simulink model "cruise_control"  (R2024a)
settings: Solver=VariableStepAuto  StartTime=0.0  StopTime=100  RelTol=1e-3
undefined symbols (not defined in the file): b, m

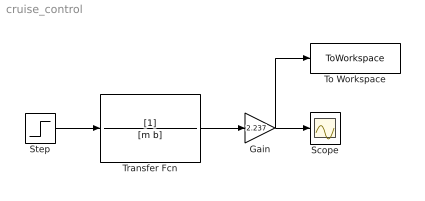
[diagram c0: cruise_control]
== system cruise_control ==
  Gain : Gain  Gain=2.237
  Scope : Scope
  Step : Step  Time=0  After=u  SampleTime=0
  To Workspace : ToWorkspace  VariableName=speed  SaveFormat=Timeseries  SampleTime=-1
  Transfer Fcn : TransferFcn  Denominator=[m b]
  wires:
  Step/1 -> Transfer Fcn/1
  Gain/1 -> To Workspace/1, Scope/1
  Transfer Fcn/1 -> Gain/1
